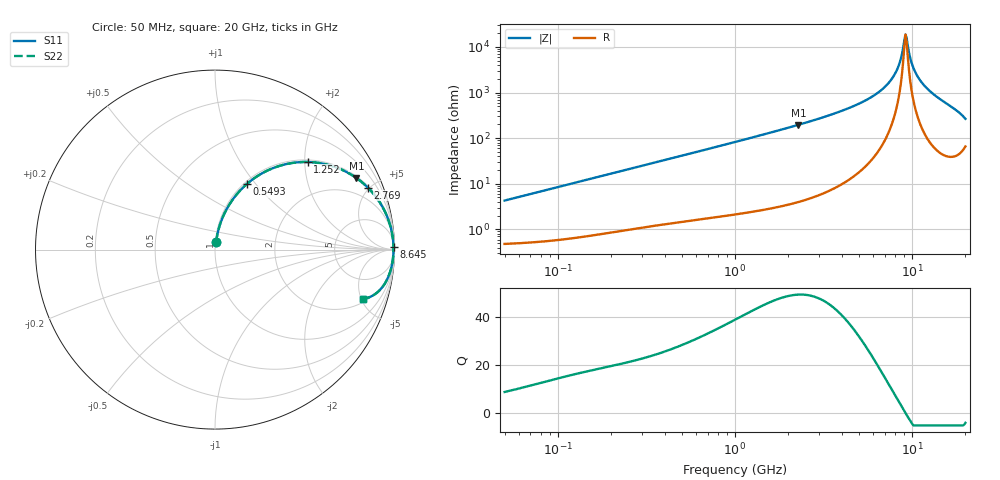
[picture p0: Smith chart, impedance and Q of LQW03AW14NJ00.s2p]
!Murata Part Number: LQW03AW14NJ00
!These Parameters are Measured in Series Mode Connection
!  o--[Z]--o
!Port1  Port2
!  o-------o
!Freq. Start=50[MHz] Stop=20[GHz], 401[Steps]
# Hz S RI R 50
!Freq.(Hz) S11(Real) S11(Imag) S21(Real) S21(Imag) S12(Real) S12(Imag) S22(Real) S22(Imag)
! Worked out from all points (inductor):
!   401 points, 50 MHz to 20 GHz, reference 50 ohm
!   read as one part in series: L = 13.5 nH near 51.52 MHz
!   highest Q = 49.2 at 2.279 GHz (marker M1), where L = 13.7 nH
!   self-resonance near 9.178 GHz
!   S11 on the Smith chart (normalised r, x): 50 MHz: 1.01, +0.09; 549.3 MHz: 1.03, +0.90; 1.252 GHz: 1.05, +2.07; 2.769 GHz: 1.10, +4.90; 8.645 GHz: open; 20 GHz: 2.31, -5.14
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5e7  0.00656 0.0421  0.9934 -0.0421  0.9934 -0.0421  0.00656 0.0421
1.364002e8  0.0196 0.1121  0.9804 -0.1121  0.9804 -0.1121  0.0196 0.1121
3.721004e8  0.0957 0.2748  0.9043 -0.2748  0.9043 -0.2748  0.0957 0.2748
5.492803e8  0.1777 0.3657  0.8223 -0.3657  0.8223 -0.3657  0.1777 0.3657
1e9  0.4056 0.4783  0.5944 -0.4783  0.5944 -0.4783  0.4056 0.4783
1.251922e9  0.5161 0.4881  0.4839 -0.4881  0.4839 -0.4881  0.5161 0.4881
2.279204e9  0.7882 0.3986  0.2118 -0.3986  0.2118 -0.3986  0.7882 0.3986
2.728004e9  0.8477 0.3492  0.1523 -0.3492  0.1523 -0.3492  0.8477 0.3492
2.769174e9  0.8521 0.3448  0.1479 -0.3448  0.1479 -0.3448  0.8521 0.3448
5.194772e9  0.9687 0.1583  0.0313 -0.1583  0.0313 -0.1583  0.9687 0.1583
6.406762e9  0.9849 0.0992  0.0151 -0.0992  0.0151 -0.0992  0.9849 0.0992
7.442007e9  0.9915 0.0581  0.00846 -0.0581  0.00846 -0.0581  0.9915 0.0581
8.141811e9  0.9938 0.0335  0.00624 -0.0335  0.00624 -0.0335  0.9938 0.0335
8.644534e9  0.9945 0.0171  0.00547 -0.0171  0.00547 -0.0171  0.9945 0.0171
9.041845e9  0.9947 0.00479  0.00527 -0.00479  0.00527 -0.00479  0.9947 0.00479
9.316812e9  0.9947 -0.00348  0.00532 0.00348  0.00532 0.00348  0.9947 -0.00348
9.892087e9  0.9941 -0.0201  0.00587 0.0201  0.00587 0.0201  0.9941 -0.0201
1.019291e10  0.9936 -0.0286  0.00638 0.0286  0.00638 0.0286  0.9936 -0.0286
1.149051e10  0.9898 -0.063  0.0102 0.063  0.0102 0.063  0.9898 -0.063
1.334722e10  0.9802 -0.1091  0.0198 0.1091  0.0198 0.1091  0.9802 -0.1091
1.670968e10  0.9447 -0.1918  0.0553 0.1918  0.0553 0.1918  0.9447 -0.1918
2e10  0.8226 -0.275  0.1774 0.275  0.1774 0.275  0.8226 -0.275
